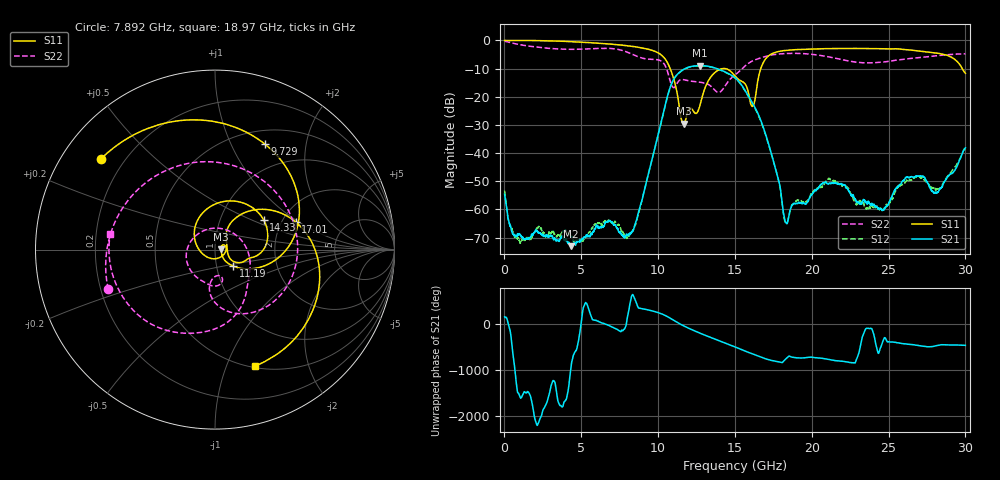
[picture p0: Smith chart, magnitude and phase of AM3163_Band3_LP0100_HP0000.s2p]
!Agilent Technologies,E8364B,MY43040894,A.07.50.67
!Agilent E8364B: A.07.50.67
!Date: Thursday, August 20, 2020 12:14:04
!Correction: S11(Full 2 Port(1,2))
!S21(Full 2 Port(1,2))
!S12(Full 2 Port(1,2))
!S22(Full 2 Port(1,2))
!S2P File: Measurements: S11, S21, S12, S22:
# Hz S  dB  R 50
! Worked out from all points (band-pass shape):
!   3201 points, 10 MHz to 30 GHz, reference 50 ohm
!   highest |S21| = -8.94 dB at 12.73 GHz (marker M1); lowest = -73.0 dB at 4.302 GHz (marker M2)
!   |S21| within 3 dB of the highest: 11.27 GHz to 14.64 GHz (3.374 GHz wide, 26 % of centre)
!   lowest |S11| = -29.6 dB at 11.66 GHz (marker M3), VSWR 1.07, Z = 53.4 + j0.284 ohm
!   |S11| at or under -10 dB: 10.79 GHz to 14.18 GHz (3.394 GHz wide, 27.2 % of centre); 14.39 GHz to 16.68 GHz (2.295 GHz wide, 14.8 % of centre); 29.8 GHz to end of sweep
!   |S22| runs from -18.5 to -0.3 dB; largest |S21 - S12| = 0.0044
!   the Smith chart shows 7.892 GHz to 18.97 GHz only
!   S11 on the Smith chart (normalised r, x): 7.892 GHz: 0.12, +0.34; 9.729 GHz: 0.66, +1.35; 11.19 GHz: 1.20, -0.22; 14.33 GHz: 1.60, +0.60; 17.01 GHz: 2.37, +0.94; 18.97 GHz: 0.51, -1.26
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1e7  -0.01 -2.1  -54.61 143.6  -53.28 -59.4  -0.28 -6.7
9.753031e8  -0.01 -26.7  -68.70 -109.9  -70.94 39.7  -1.46 -82.6
2.156159e9  -0.06 -59.2  -67.77 -25.1  -66.41 -19.1  -2.41 -159.9
4.302319e9  -0.41 -116.7  -73.02 63.1  -69.17 178.4  -3.15 85.9
5.014581e9  -0.61 -135.6  -70.90 63.1  -70.83 -136.0  -3.11 47.1
6.870212e9  -1.27 173.2  -64.02 -54.6  -64.29 -69.1  -2.82 -72.8
7.891747e9  -1.81 141.6  -69.41 -65.0  -69.73 -31.0  -3.95 -159.5
9.728634e9  -3.74 64.8  -39.49 -97.2  -39.60 -97.8  -6.72 5.4
1.000979e10  -4.43 47.6  -33.26 -125.3  -33.39 -126.1  -6.91 -25.3
1.119065e10  -17.36 -42.4  -12.41 33.1  -12.46 33.2  -15.66 -75.7
1.165924e10  -29.56 4.6  -10.28 -49.3  -10.37 -49.4  -13.91 -95.6
1.272763e10  -22.95 -158.7  -8.94 151.4  -8.99 151.6  -14.82 -131.8
1.433022e10  -9.96 31.7  -11.09 -55.9  -11.17 -55.6  -16.35 23.2
1.5005e10  -12.59 -8.5  -13.25 -144.4  -13.33 -144.3  -12.27 -39.1
1.614837e10  -23.38 10.2  -22.25 63.9  -22.48 64.0  -7.26 -87.3
1.701058e10  -6.46 18.8  -33.51 -42.8  -33.78 -40.4  -5.65 -120.0
1.828516e10  -3.53 -47.9  -64.34 -52.4  -64.60 -76.7  -4.63 -164.9
1.89693e10  -3.26 -71.2  -57.87 -20.0  -57.15 -18.3  -4.58 171.8
2.000958e10  -3.02 -100.1  -54.78 -5.8  -54.52 -10.2  -4.92 134.7
2.266182e10  -2.83 -161.3  -54.76 -126.3  -55.70 -129.7  -7.54 16.9
2.500479e10  -3.00 144.2  -57.75 -33.0  -57.95 -42.9  -7.44 -95.8
3e10  -11.67 -29.0  -38.12 -111.7  -37.81 -116.2  -4.74 100.8
